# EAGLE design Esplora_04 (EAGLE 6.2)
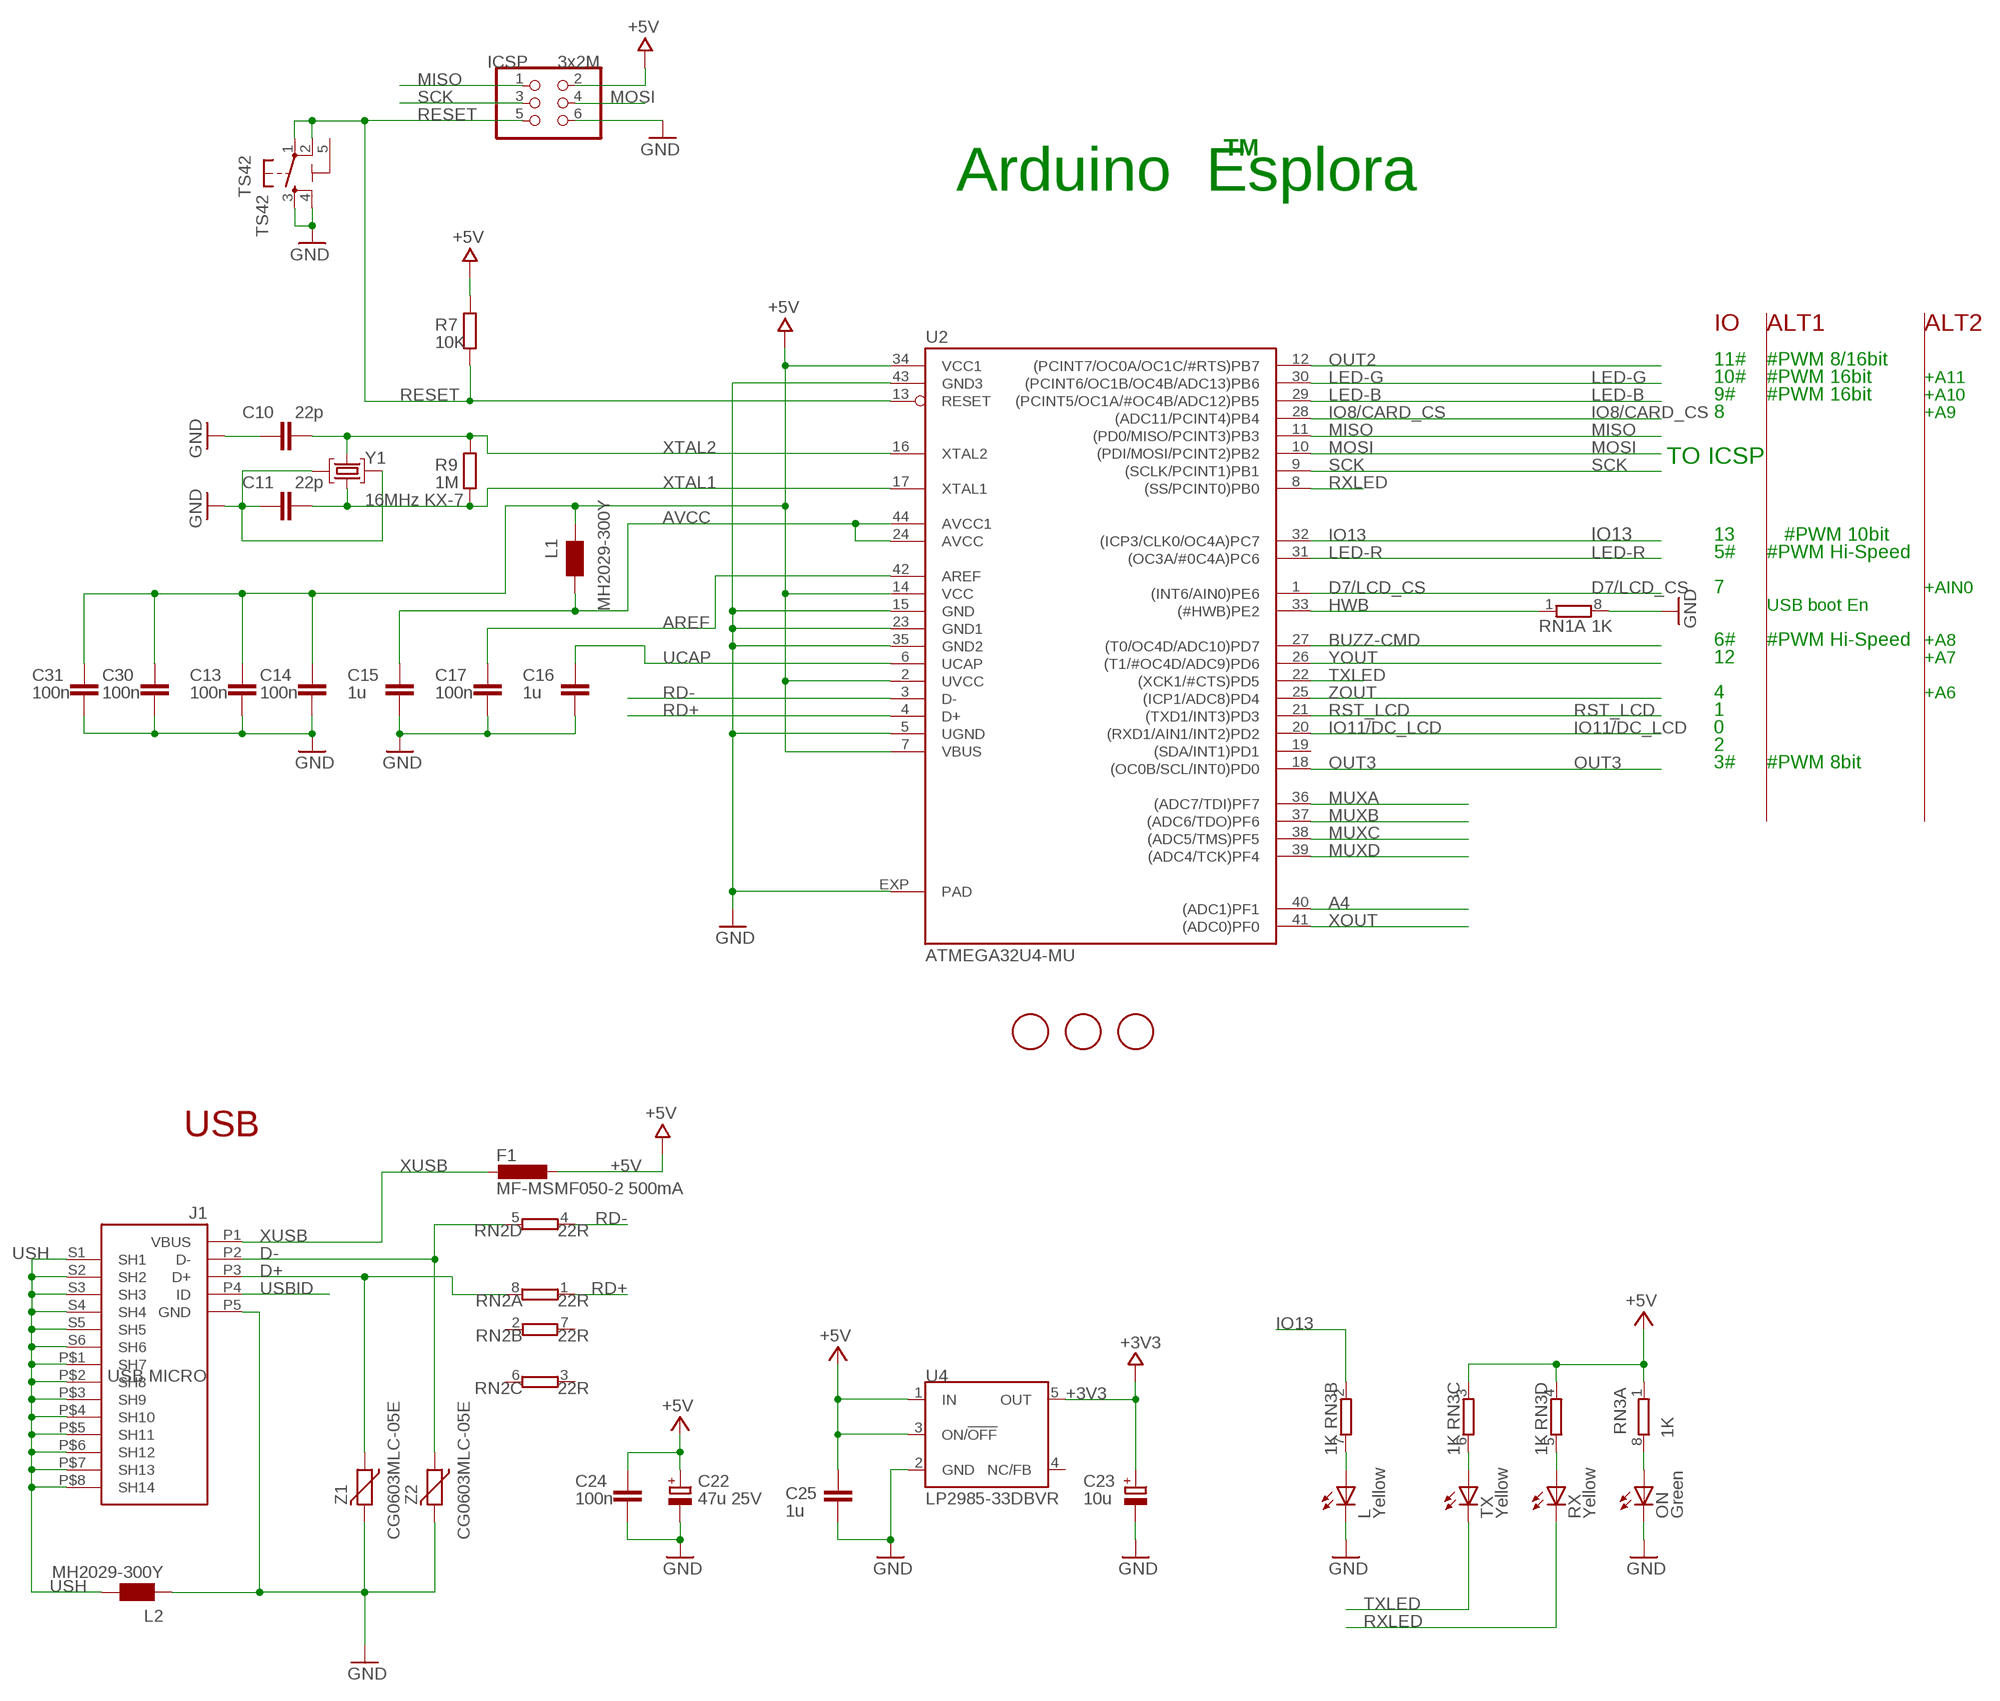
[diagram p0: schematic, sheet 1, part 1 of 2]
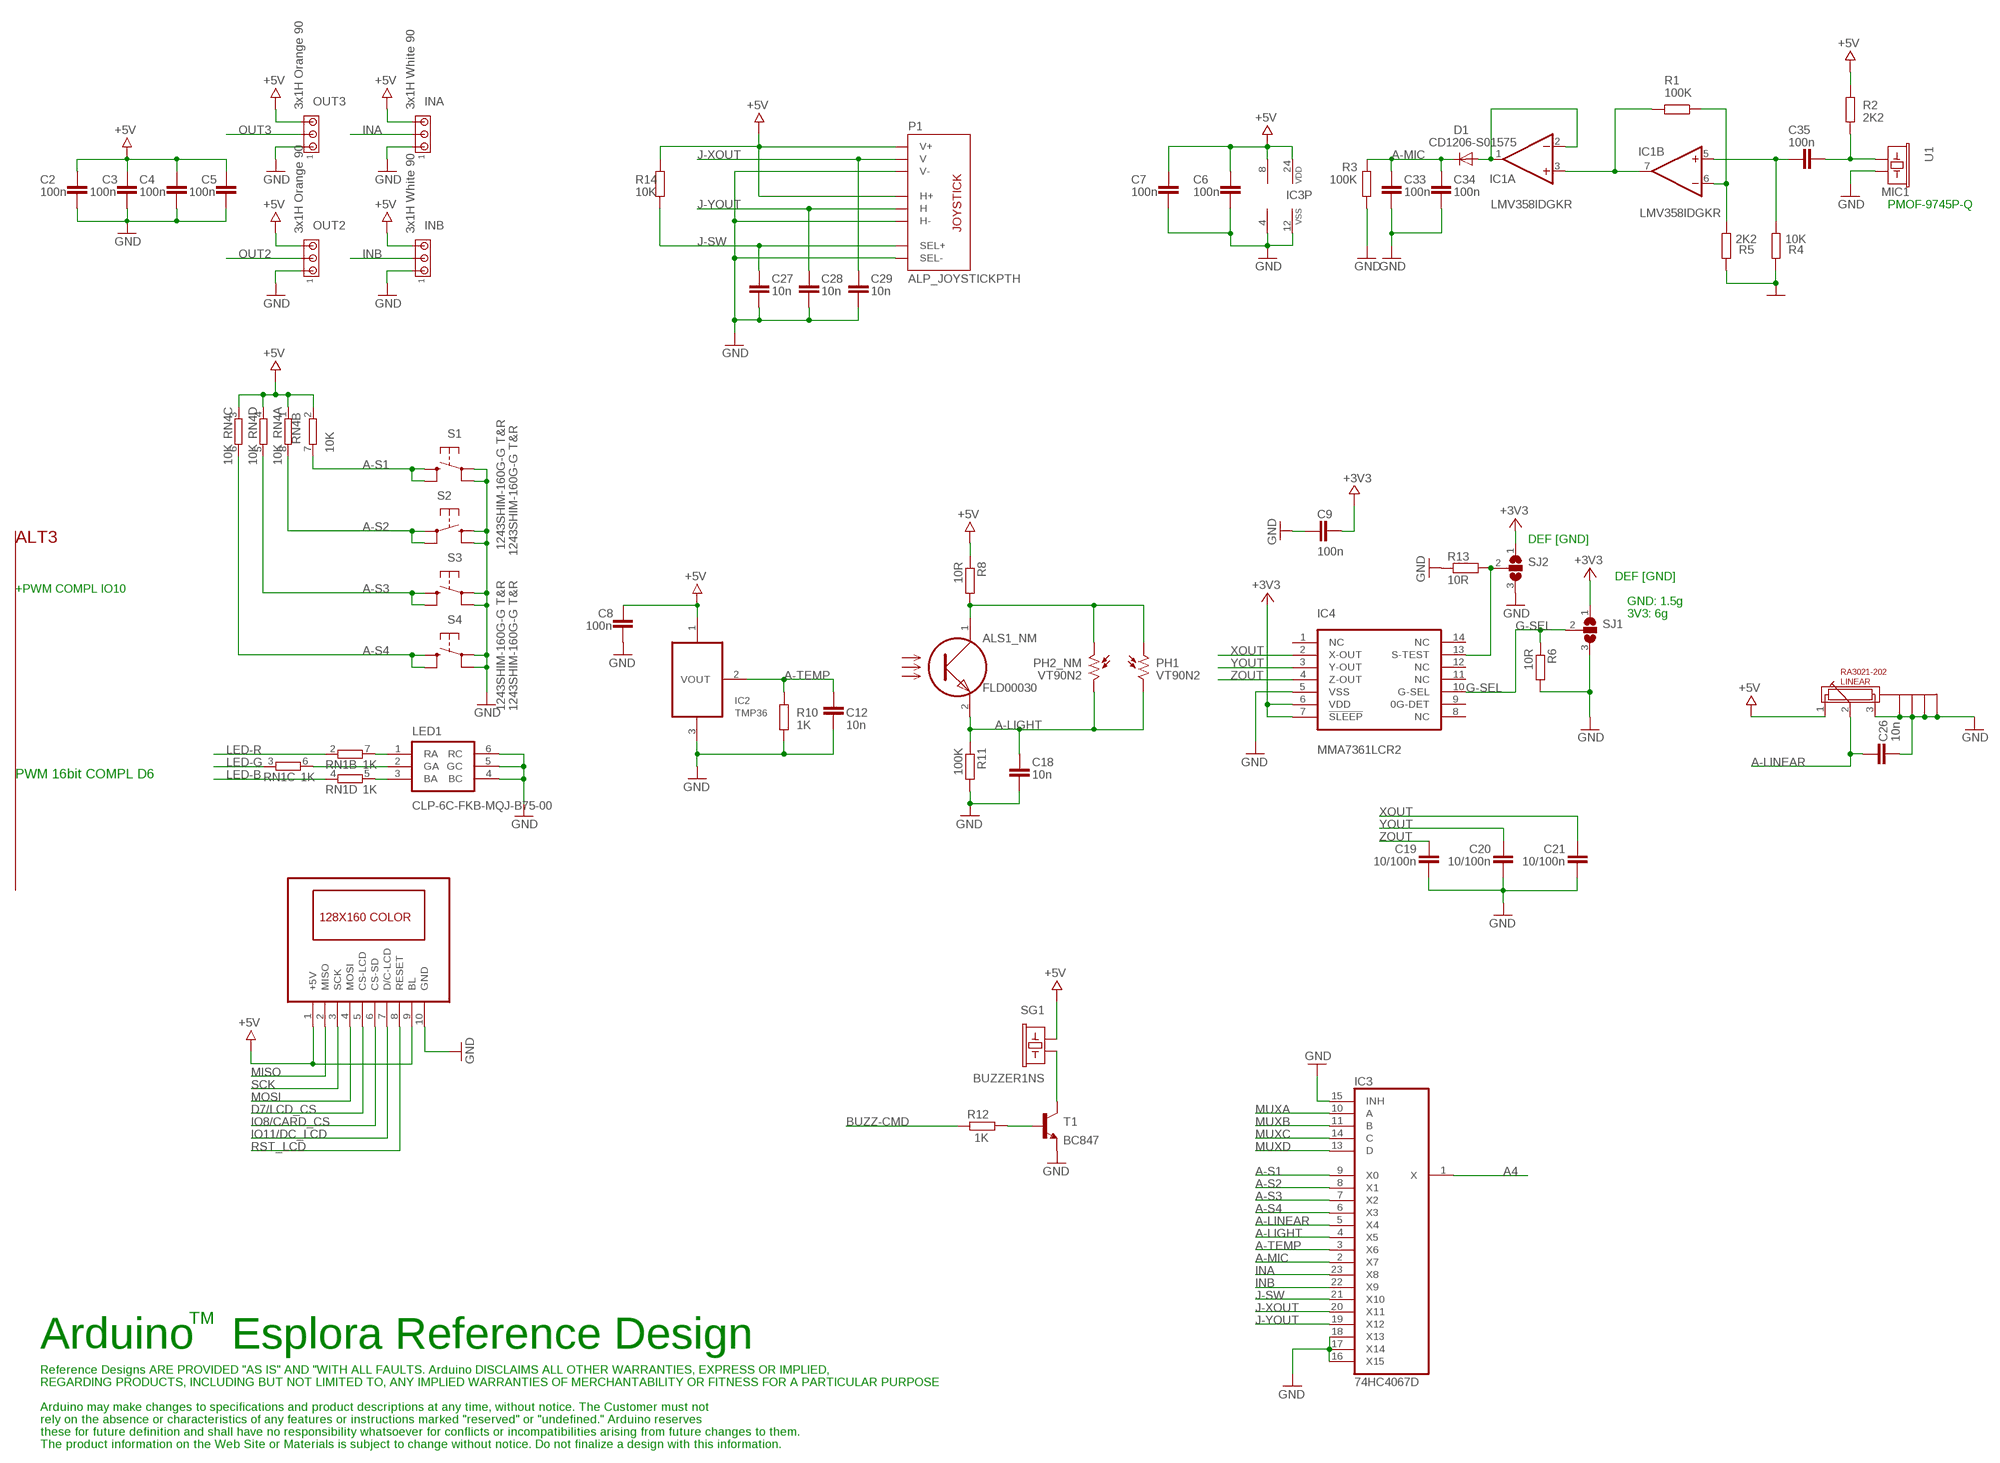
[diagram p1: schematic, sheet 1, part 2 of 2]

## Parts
ALS1_NM  FLD00030  [FLD00030]
C2  100n  C-EUC0603  [C0603-ROUND]
C3  100n  C-EUC0603  [C0603-ROUND]
C4  100n  C-EUC0603  [C0603-ROUND]
C5  100n  C-EUC0603  [C0603-ROUND]
C6  100n  C-EUC0603  [C0603-ROUND]
C7  100n  C-EUC0603  [C0603-ROUND]
C8  100n  C-EUC0603  [C0603-ROUND]
C9  100n  C-EUC0603  [C0603-ROUND]
C10  22p  C-EUC0603  [C0603-ROUND]
C11  22p  C-EUC0603  [C0603-ROUND]
C12  10n  C-EUC0603  [C0603-ROUND]
C13  100n  C-EUC0603  [C0603-ROUND]
C14  100n  C-EUC0603  [C0603-ROUND]
C15  1u  C-EUC0603  [C0603-ROUND]
C16  1u  C-EUC0603  [C0603-ROUND]
C17  100n  C-EUC0603  [C0603-ROUND]
C18  10n  C-EUC0603  [C0603-ROUND]
C19  10/100n  C-EUC0603  [C0603-ROUND]
C20  10/100n  C-EUC0603  [C0603-ROUND]
C21  10/100n  C-EUC0603  [C0603-ROUND]
C22  47u 25V  CPOL-EUD  [PANASONIC_D]
C23  10u  CPOL-EUSMCB  [SMC_B]
C24  100n  C-EUC0603  [C0603-ROUND]
C25  1u  C-EUC0603  [C0603-ROUND]
C26  10n  C-EUC0603  [C0603-ROUND]
C27  10n  C-EUC0603  [C0603-ROUND]
C28  10n  C-EUC0603  [C0603-ROUND]
C29  10n  C-EUC0603  [C0603-ROUND]
C30  100n  C-EUC0603  [C0603-ROUND]
C31  100n  C-EUC0603  [C0603-ROUND]
C33  100n  C-EUC0603  [C0603-ROUND]
C34  100n  C-EUC0603  [C0603-ROUND]
C35  100n  C-EUC0603  [C0603-ROUND]
D1  CD1206-S01575  DIODE-MINIMELF  [MINIMELF]
F1  MF-MSMF050-2 500mA  L-EUL1812  [L1812]
FID1  FIDUCIALMOUNT  [FIDUCIA-MOUNT]
FID2  FIDUCIALMOUNT  [FIDUCIA-MOUNT]
FID3  FIDUCIALMOUNT  [FIDUCIA-MOUNT]
IC1  LMV358IDGKR  LMV358MMX  [MSOP08]
IC2  TMP36  LM35TO-92  [TO92]
IC3  74HC4067D  4067D  [SO24W]
IC4  MMA7361LCR2  MMA7361LC  [LGA-14_3X5/0.8]
ICSP  3x2M  PINHD-2X3  [2X03]
INA  3x1H White 90  MTA03-100  [10X03MTA]
INB  3x1H White 90  MTA03-100  [10X03MTA]
J1  USB MICRO  MYCON2_USB-MINI-B  [CON2_USB_MICRO_B_AT]
L  Yellow  LEDCHIPLED_0805  [CHIPLED_0805]
L1  MH2029-300Y  WE-CBF_0805  [0805]
L2  MH2029-300Y  WE-CBF_0805  [0805]
LCD1  LCD1  1.8'_LCD-TFT(128X160)+SD-CARD  [1.8'_LCD-LCD-TFT(128X160)]
LED1  CLP-6C-FKB-MQJ-B75-00  RGB-LED  [RGB-LED]
LINEAR  RA3021-202  [RA3021-202]
ON  Green  LEDCHIPLED_0805  [CHIPLED_0805]
OUT2  3x1H Orange 90  MTA03-100  [10X03MTA]
OUT3  3x1H Orange 90  MTA03-100  [10X03MTA]
P1  ALP_JOYSTICKPTH  [ALP_JOYSTICK]
PH1  VT90N2  A1050_09  [T0-46-A10XX]
PH2_NM  VT90N2  B1060_23  [TO-8_B10]
R1  100K  R-EU_R0603  [R0603-ROUND]
R2  2K2  R-EU_R0603  [R0603-ROUND]
R3  100K  R-EU_R0603  [R0603-ROUND]
R4  10K  R-EU_R0603  [R0603-ROUND]
R5  2K2  R-EU_R0603  [R0603-ROUND]
R6  10R  R-EU_R0603  [R0603-ROUND]
R7  10K  R-EU_R0603  [R0603-ROUND]
R8  10R  R-EU_R0603  [R0603-ROUND]
R9  1M  R-EU_R0603  [R0603-ROUND]
R10  1K  R-EU_R0603  [R0603-ROUND]
R11  100K  R-EU_R0603  [R0603-ROUND]
R12  1K  R-EU_R0603  [R0603-ROUND]
R13  10R  R-EU_R0603  [R0603-ROUND]
R14  10K  R-EU_R1206  [R1206]
RN1  1K  4R-NCAY16  [CAY16]
RN2  22R  4R-NCAY16  [CAY16]
RN3  1K  4R-NCAY16  [CAY16]
RN4  10K  4R-NCAY16  [CAY16]
RX  Yellow  LEDCHIPLED_0805  [CHIPLED_0805]
S1  1243SHIM-160G-G T&R  TACTILE_SWITCHTACTILE_SWITCH_SMD-12MM  [TACTILE-SMD-12MM]
S2  1243SHIM-160G-G T&R  TACTILE_SWITCHTACTILE_SWITCH_SMD-12MM  [TACTILE-SMD-12MM]
S3  1243SHIM-160G-G T&R  TACTILE_SWITCHTACTILE_SWITCH_SMD-12MM  [TACTILE-SMD-12MM]
S4  1243SHIM-160G-G T&R  TACTILE_SWITCHTACTILE_SWITCH_SMD-12MM  [TACTILE-SMD-12MM]
SG1  BUZZER1NS  [BUZZER-12MM-NS]
SJ1  SJ2W  [SJ_2]
SJ2  SJ2W  [SJ_2]
T1  BC847  [SOT23]
TS42  TS42  [TS42]
TX  Yellow  LEDCHIPLED_0805  [CHIPLED_0805]
U1  MIC1  MIC9.7MM  [MIC-9.7MM]
U2  ATMEGA32U4-MU  [QFN44ML7X7]
U4  LP2985-33DBVR  LP2985-XXDBVR33  [SOT23-DBV]
Y1  16MHz KX-7  CRYSTAL-3.2-2.5  [CRYSTAL-3.2-2.5]
Z1  CG0603MLC-05E  VARISTORCN0603  [CT/CN0603]
Z2  CG0603MLC-05E  VARISTORCN0603  [CT/CN0603]

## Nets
+3V3 [power]: C9.2 C23.+ IC4.6(VDD) IC4.7(!SLEEP) SJ1.1 SJ2.1 U4.5(OUT)
+5V [power]: C2.2 C3.2 C4.2 C5.2 C6.2 C7.2 C8.2 C13.1 C14.1 C22.+ C24.2 C25.2 C30.1 C31.1 F1.1 IC1.8(P:V+) IC2.1(+VS) IC3.24(VDD) ICSP.2 INA.3 INB.3 L1.1 LCD1.1(+5V) LCD1.9(BL) LINEAR.1 OUT2.3 OUT3.3 P1.H1(H+) P1.V1(V+) R2.1 R7.1 R8.1 R14.1 RN3.1 RN3.3 RN3.4 RN4.1 RN4.2 RN4.3 RN4.4 SG1.+ U2.2(UVCC) U2.7(VBUS) U2.14(VCC) U2.34(VCC1) U4.1(IN) U4.3(ON/!OFF)
A4: IC3.1(X) U2.40((ADC1)PF1)
A-LIGHT: ALS1_NM.2 C18.2 IC3.4(X5) PH1.2 PH2_NM.2 R11.1
A-LINEAR: C26.2 IC3.5(X4) LINEAR.2
A-MIC: C33.2 C34.2 D1.C IC3.2(X7) R3.1
A-S1: IC3.9(X0) RN4.7 S1.P$3 S1.P$4
A-S2: IC3.8(X1) RN4.8 S2.P$1 S2.P$2
A-S3: IC3.7(X2) RN4.5 S3.P$3 S3.P$4
A-S4: IC3.6(X3) RN4.6 S4.P$3 S4.P$4
A-TEMP: C12.2 IC2.2(VOUT) IC3.3(X6) R10.1
AREF [aref]: C17.2 U2.42(AREF)
AVCC: C15.1 L1.2 U2.24(AVCC) U2.44(AVCC1)
BUZZ-CMD: R12.2 U2.27((T0/OC4D/ADC10)PD7)
D7/LCD_CS: LCD1.5(CS-LCD) U2.1((INT6/AIN0)PE6)
D+: J1.P3(D+) RN2.8 Z1.1
D-: J1.P2(D-) RN2.5 Z2.1
G-SEL: IC4.10(G-SEL) R6.1 SJ1.2
GND [gnd]: C2.1 C3.1 C4.1 C5.1 C6.1 C7.1 C8.1 C9.1 C10.1 C11.2 C12.1 C13.2 C14.2 C15.2 C16.2 C17.1 C18.1 C19.1 C20.1 C21.1 C22.- C23.- C24.1 C25.1 C26.1 C27.1 C28.1 C29.1 C30.2 C31.2 C33.1 C34.1 IC1.4(P:V-) IC2.3(GND) IC3.12(VSS) IC3.15(INH) IC3.16(X15) IC3.17(X14) IC3.18(X13) IC4.5(VSS) ICSP.6 INA.1 INB.1 J1.P5(GND) L2.1 L.C LCD1.10(GND) LED1.4(BC) LED1.5(GC) LED1.6(RC) LINEAR.3 LINEAR.CHASSIS1(CHASSIS-GND-1) LINEAR.CHASSIS2(CHASSIS-GND-2) LINEAR.CHASSIS3(CHASSIS-GND-3) LINEAR.CHASSIS4(CHASSIS-GND-4) ON.C OUT2.1 OUT3.1 P1.B2A(SEL-) P1.H3(H-) P1.V3(V-) R3.2 R4.2 R5.2 R6.2 R10.2 R11.2 R13.1 RN1.8 S1.P$1 S1.P$2 S2.P$3 S2.P$4 S3.P$1 S3.P$2 S4.P$1 S4.P$2 SJ1.3 SJ2.3 T1.2(E) TS42.3 TS42.4 U1.2 U2.5(UGND) U2.15(GND) U2.23(GND1) U2.35(GND2) U2.43(GND3) U2.EXP(PAD) U4.2(GND) Y1.2(GND) Y1.4(GND) Z1.2 Z2.2
HWB: RN1.1 U2.33((#HWB)PE2)
INA: IC3.23(X8) INA.2
INB: IC3.22(X9) INB.2
IO8/CARD_CS: LCD1.6(CS-SD) U2.28((ADC11/PCINT4)PB4)
IO11/DC_LCD: LCD1.7(D/C-LCD) U2.20((RXD1/AIN1/INT2)PD2)
IO13: RN3.2 U2.32((ICP3/CLK0/OC4A)PC7)
J-SW: C27.2 IC3.21(X10) P1.B1A(SEL+) R14.2
J-XOUT: C29.2 IC3.20(X11) P1.V2(V)
J-YOUT: C28.2 IC3.19(X12) P1.H2(H)
LED-B: RN1.4 U2.29((PCINT5/OC1A/#OC4B/ADC12)PB5)
LED-G: RN1.3 U2.30((PCINT6/OC1B/OC4B/ADC13)PB6)
LED-R: RN1.2 U2.31((OC3A/#0C4A)PC6)
MISO: ICSP.1 LCD1.2(MISO) U2.11((PD0/MISO/PCINT3)PB3)
MOSI: ICSP.4 LCD1.4(MOSI) U2.10((PDI/MOSI/PCINT2)PB2)
MUXA: IC3.10(A) U2.36((ADC7/TDI)PF7)
MUXB: IC3.11(B) U2.37((ADC6/TDO)PF6)
MUXC: IC3.14(C) U2.38((ADC5/TMS)PF5)
MUXD: IC3.13(D) U2.39((ADC4/TCK)PF4)
N$1: D1.A IC1.1(A:OUT) IC1.2(A:-IN)
N$2: L.A RN3.7
N$3: ON.A RN3.8
N$4: IC4.13(S-TEST) R13.2 SJ2.2
N$6: RN3.6 TX.A
N$8: RN3.5 RX.A
N$11: LED1.1(RA) RN1.7
N$12: LED1.2(GA) RN1.6
N$13: LED1.3(BA) RN1.5
N$17: SG1.- T1.3(C)
N$19: C35.1 R2.2 U1.1
N$20: C35.2 IC1.5(B:+IN) R4.1
N$21: IC1.6(B:-IN) R1.1 R5.1
N$23: IC1.3(A:+IN) IC1.7(B:OUT) R1.2
N$27: ALS1_NM.1 PH1.1 PH2_NM.1 R8.2
N$31: R12.1 T1.1(B)
OUT2: OUT2.2 U2.12((PCINT7/OC0A/OC1C/#RTS)PB7)
OUT3: OUT3.2 U2.18((OC0B/SCL/INT0)PD0)
RD+: RN2.1 U2.4(D+)
RD-: RN2.4 U2.3(D-)
RESET: ICSP.5 R7.2 TS42.1 TS42.2 U2.13(RESET)
RST_LCD: LCD1.8(RESET) U2.21((TXD1/INT3)PD3)
RXLED: RX.C U2.8((SS/PCINT0)PB0)
SCK: ICSP.3 LCD1.3(SCK) U2.9((SCLK/PCINT1)PB1)
TXLED: TX.C U2.22((XCK1/#CTS)PD5)
UCAP: C16.1 U2.6(UCAP)
USBID: J1.P4(ID)
USH [gnd]: J1.P$1(SH7) J1.P$2(SH8) J1.P$3(SH9) J1.P$4(SH10) J1.P$5(SH11) J1.P$6(SH12) J1.P$7(SH13) J1.P$8(SH14) J1.S1(SH1) J1.S2(SH2) J1.S3(SH3) J1.S4(SH4) J1.S5(SH5) J1.S6(SH6) L2.2
XOUT: C21.2 IC4.2(X-OUT) U2.41((ADC0)PF0)
XTAL1: C11.1 R9.1 U2.17(XTAL1) Y1.1(C1)
XTAL2: C10.2 R9.2 U2.16(XTAL2) Y1.3(C2)
XUSB [usbvcc]: F1.2 J1.P1(VBUS)
YOUT: C20.2 IC4.3(Y-OUT) U2.26((T1/#OC4D/ADC9)PD6)
ZOUT: C19.2 IC4.4(Z-OUT) U2.25((ICP1/ADC8)PD4)
Unconnected: IC4.1(NC) IC4.8(NC) IC4.9(0G-DET) IC4.11(NC) IC4.12(NC) IC4.14(NC) RN2.2 RN2.3 RN2.6 RN2.7 U2.19((SDA/INT1)PD1) U4.4(NC/FB)

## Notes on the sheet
- PMOF-9745P-Q
- TM
- Arduino  Esplora
- IO | ALT1 | ALT2 | ALT3 | DEF [GND]
- 11# | #PWM 8/16bit
- 10# | #PWM 16bit | +A11 | DEF [GND]
- 9# | #PWM 16bit | +A10 | +PWM COMPL IO10
- 8 | +A9 | GND: 1.5g
- 3V3: 6g
- TO ICSP
- 13 | #PWM 10bit
- 5# | #PWM Hi-Speed
- 7 | +AIN0
- USB boot En
- 6# | #PWM Hi-Speed | +A8
- 12 | +A7 | PWM 16bit COMPL D6
- 4 | +A6
- 1
- 0
- 2
- 3# | #PWM 8bit
- USB
- TM
- Arduino   Esplora Reference Design
- Reference Designs ARE PROVIDED "AS IS" AND "WITH ALL FAULTS. Arduino DISCLAIMS ALL OTHER WARRANTIES, EXPRESS OR IMPLIED,
- REGARDING PRODUCTS, INCLUDING BUT NOT LIMITED TO, ANY IMPLIED WARRANTIES OF MERCHANTABILITY OR FITNESS FOR A PARTICULAR PURPOSE
- Arduino may make changes to specifications and product descriptions at any time, without notice. The Customer must not
- rely on the absence or characteristics of any features or instructions marked "reserved" or "undefined." Arduino reserves
- these for future definition and shall have no responsibility whatsoever for conflicts or incompatibilities arising from future changes to them.
- The product information on the Web Site or Materials is subject to change without notice. Do not finalize a design with this information.

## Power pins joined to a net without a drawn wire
5-GND: TS42.5(5-GND)

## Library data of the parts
ALS1_NM = SmartPrj:FLD00030: FLD00030 Analog Ambient Light Sensor FAIRCHILD Semiconductor
C2-C21 C24-C31 C33-C35 = SmartPrj:C-EU: CAPACITOR, European symbol
C22 C23 = rcl:CPOL-EU: POLARIZED CAPACITOR, European symbol
D1 = diode:DIODE-: DIODE
F1 = rcl:L-EU: INDUCTOR, European symbol
FID1-FID3 = SmartPrj:FIDUCIALMOUNT
IC1 = linear:LMV358?*: Dual General Purpose, Low Voltage, Rail-to-Rail Output Operational Amplifiers Source: http://www.national.com/mpf/LM/LMV321.html http://www.national.com/dt/lmv_qual.pdf
IC2 = SmartPrj:LM35: LM35 Precision Centigrade Temperature Sensors
IC3 = 40xx:4067: 16-channel ANALOG MULTIPLEXER
IC4 = SmartPrj:MMA7361LC: MMA7361LC Three Axis Accelerometer Freescale Semiconductor
ICSP = SmartPrj:PINHD-2X3: PIN HEADER
INA INB OUT2 OUT3 = con-amp:MTA03-100: AMP connector
J1 = SmartPrj:MYCON2_USB-MINI-B
L ON RX TX = led:LED: LED
L1 L2 = wuerth-elektronik:WE-CBF: SMD EMI Suppression Ferrite Beads
LCD1 = SmartPrj:1.8'_LCD-TFT(128X160)+SD-CARD: 1.8Inch LCD Display + SD Card SmartProjects.it
LED1 = SmartPrj:RGB-LED: CREE RGB-LED/PLCC6-SMD
LINEAR = st-mod v1.1:RA3021-202: RA3021-202 Linear Potentiometer P.C.B. single unit case-earthing mounting type Travel: 30mm
P1 = tinker_it:ALP_JOYSTICK: Thumb Joystick Joystick commonly found in PS2 controllers. Two pots and a select switch. Footprint proven. Spark Fun Electronics SKU : COM-09032
PH1 = photo-elements:A10: Sensor Robust Light Sensing Applications
PH2_NM = photo-elements:?1060*: Sensor Street Light control
R1-R14 = SmartPrj:R-EU_: RESISTOR, European symbol
RN1-RN4 = resistor-dil:4R-N: Array Chip Resistor Source: RS Component / Phycomp; OC_FARNELL: unknown; OC_NEWARK: unknown
S1-S4 = SmartPrj:TACTILE_SWITCH: Momentary Switch Button commonly used for reset or general input.
SG1 = SmartPrj:BUZZER1: Buzzer 12-22mm
SJ1 SJ2 = jumper:SJ2W: SMD solder JUMPER
T1 = transistor:BC847: NPN TRANSISTOR
TS42 = SmartPrj:TS42: TS42 Dongnan Electronics Tact switch VDC 12V - 50mA
U1 = SparkFun:MIC: Microphone
U2 = SmartPrj:ATMEGA32U4-
U4 = SmartPrj:LP2985-XXDBVR: ULTRALOW-POWER 50-mA LOW-DROPOUT LINEAR REGULATORS 50-mA Low-Dropout Regulator Source: http://focus.ti.com/lit/ds/symlink/tps77001.pdf
Y1 = SmartPrj:CRYSTAL-3.2-2.5
Z1 Z2 = varistor:VARISTOR: VARISTOR

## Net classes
0 default: width 0.254 mm, drill 0.61 mm, clearance 0.254 mm
1 power: width 0.254 mm, drill 0.61 mm, clearance 0.254 mm
2 gnd: width 0.254 mm, drill 0.61 mm, clearance 0.254 mm
3 usbvcc: width 0.254 mm, drill 0.61 mm, clearance 0.254 mm
4 aref: width 0.254 mm, drill 0.61 mm, clearance 0.254 mm

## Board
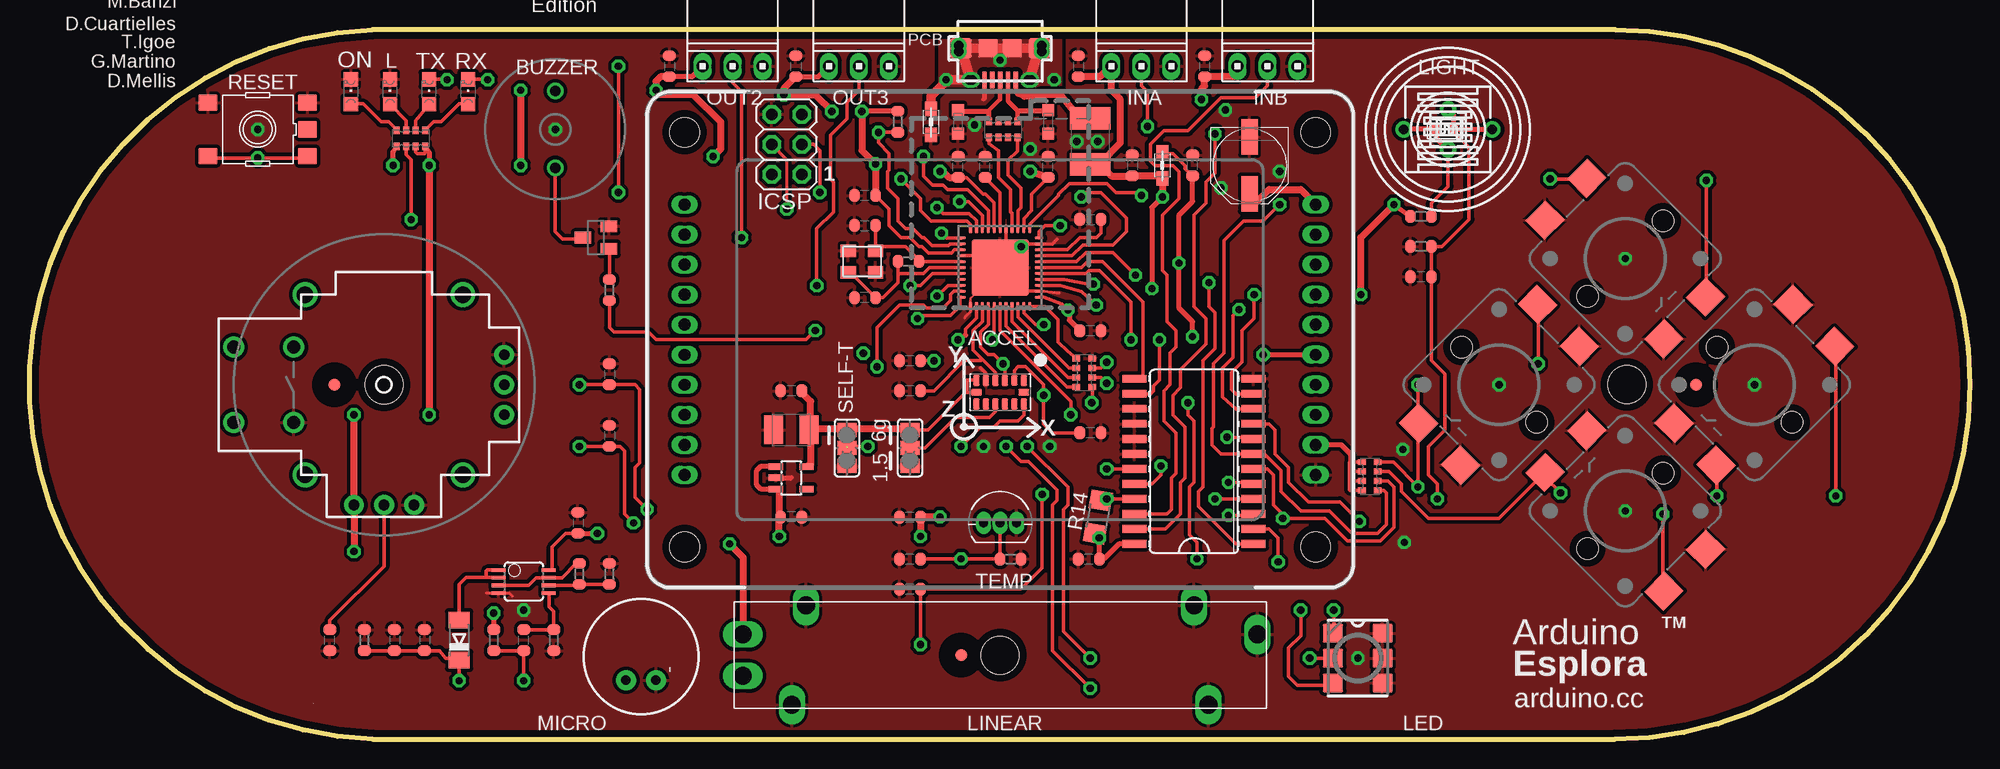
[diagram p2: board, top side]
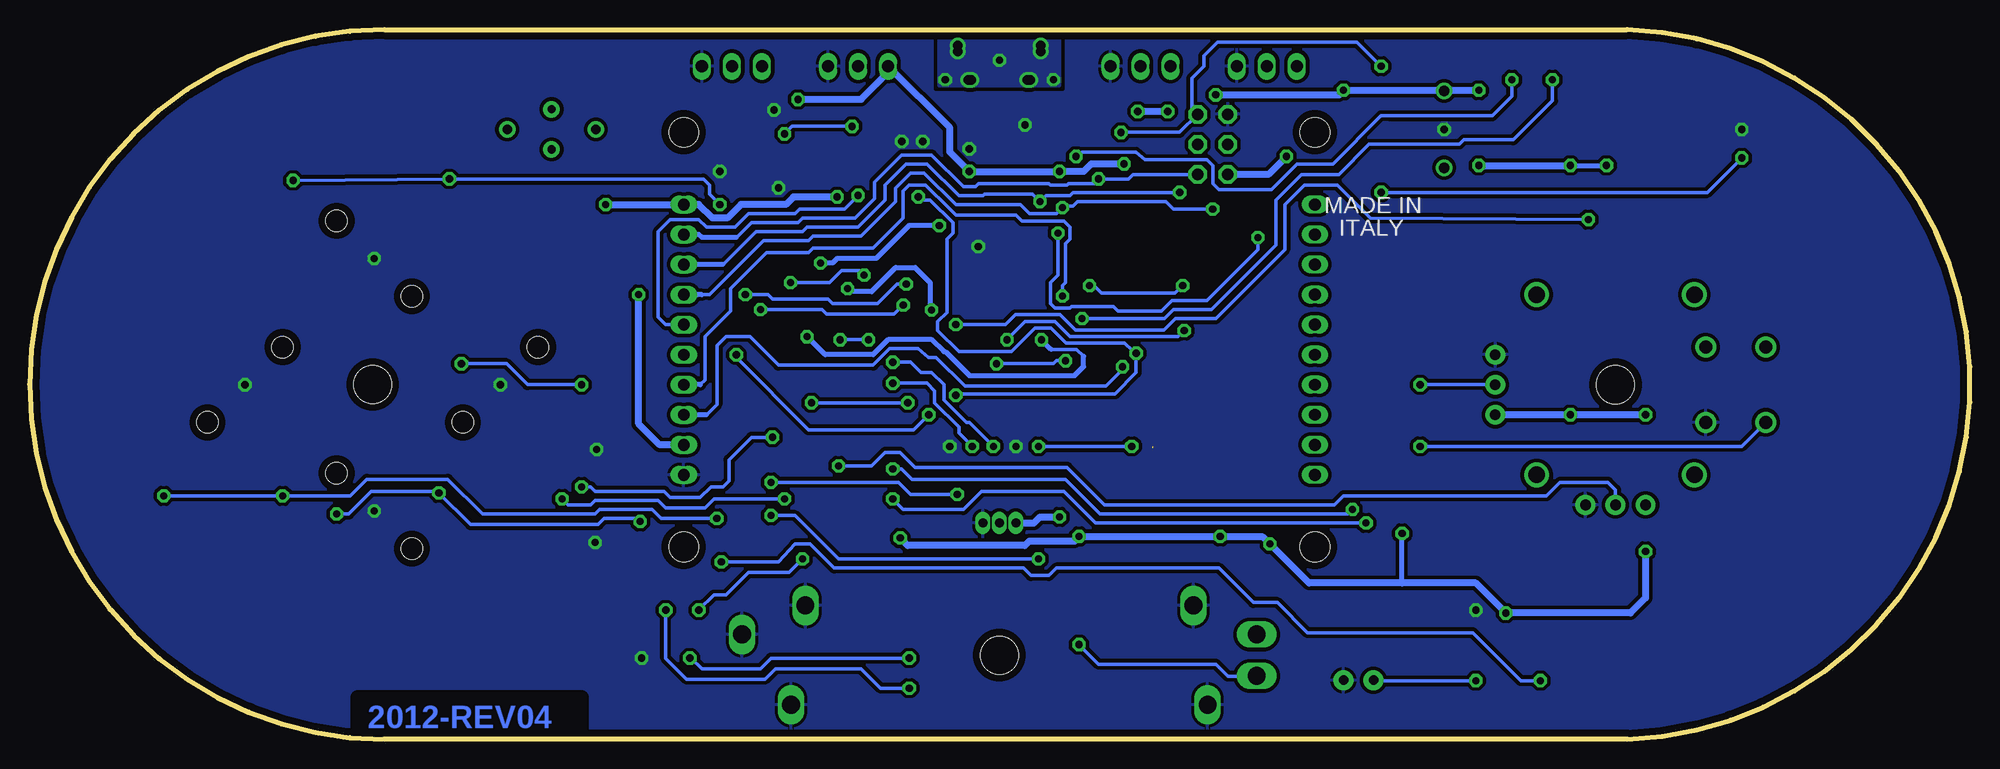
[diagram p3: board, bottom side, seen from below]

Size 163.98 x 60 mm. Coordinates in mm from the lower left corner, seen from the top.
Outline: 28.98,0 133.98,0 arc180 133.98,60 28.98,60 arc176 28.98,0
Copper layers (1*16): Top 0.035mm / dielectric 1.5mm / Bottom 0.035mm
Design rules: minimum track width 10mil, minimum drill 22mil, track to track 10mil, track to pad 10mil, pad to pad 8mil, via to via 12mil, smd to smd 8mil, copper to edge 24mil, drill to drill 12mil, minimum pad ring 10mil, minimum via ring 10mil, stop-mask expansion 2mil, vias tented up to drill 30mil, thermal gap 10mil
Holes 3.2 mm at 82.02,7.11 29.95,29.97 134.98,30
bRestrict: 3 lines
vRestrict: area 47.9,10.3 to 48.5,10.8; area 50.4,10.2 to 50.9,11

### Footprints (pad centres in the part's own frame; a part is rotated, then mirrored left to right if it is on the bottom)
FLD00030 = smd 0.8 x 0.9: 1 -0.75,0; 2 0.75,0
C0603-ROUND = smd 0.898 x 1.1: 1 -0.889,0; 2 0.889,0
PANASONIC_D = smd 3 x 1.4: + 2.4,0; - -2.4,0
SMC_B = smd 1.6 x 2.4: + -1.5,0; - 1.5,0
MINIMELF = smd 1.4 x 1.8: A 1.7,0; C -1.7,0
L1812 = smd 1.9 x 3.4: 1 -1.95,0; 2 1.95,0
FIDUCIA-MOUNT = smd 1.016 x 1.016: P$1 0,0
MSOP08 = smd 0.3 x 1.2: 1 -0.976,-2.113; 2 -0.326,-2.113; 3 0.324,-2.113; 4 0.974,-2.113; 5 0.974,2.112; 6 0.324,2.112; 7 -0.326,2.112; 8 -0.976,2.112
TO92 = drill 0.75 pad 1.092 long: 1 -1.397,0; 2 0,0; 3 1.397,0
SO24W = smd 0.66 x 2.032: 1 -6.985,-5.029; 2 -5.715,-5.029; 3 -4.445,-5.029; 4 -3.175,-5.029; 5 -1.905,-5.029; 6 -0.635,-5.029; 7 0.635,-5.029; 8 1.905,-5.029; 9 3.175,-5.029; 10 4.445,-5.029; 11 5.715,-5.029; 12 6.985,-5.029; 13 6.985,5.029; 14 5.715,5.029; 15 4.445,5.029; 16 3.175,5.029; 17 1.905,5.029; 18 0.635,5.029; 19 -0.635,5.029; 20 -1.905,5.029; 21 -3.175,5.029; 22 -4.445,5.029; 23 -5.715,5.029; 24 -6.985,5.029
LGA-14_3X5/0.8 = smd 0.55 x 0.9: 1 -2,-1; 3 -0.4,-1; 4 0.4,-1; 5 1.2,-1; 6 2,-1; 8 2,1; 9 1.2,1; 10 0.4,1; 11 -0.4,1; 12 -1.2,1; 13 -2,1 | smd 0.55 x 0.85: 2 -1.2,-1 | smd 0.9 x 0.55: 7 2,0; 14 -2,0
2X03 = drill 0.95 pad 1.55 octagon: 1 -2.54,-1.27; 2 -2.54,1.27; 3 0,-1.27; 4 0,1.27; 5 2.54,-1.27; 6 2.54,1.27
10X03MTA = drill 1.016 long: 1 2.54,0; 2 0,0; 3 -2.54,0
CON2_USB_MICRO_B_AT = smd 0.406 x 1.346: P1 -1.321,2.692; P2 -0.66,2.692; P3 0,2.692; P4 0.66,2.692; P5 1.321,2.692 | drill 0.8 pad 1.27: P$1 -2.616,2.692 | drill 0.8 pad 1.245: P$2 -2.362,2.692; P$7 2.362,2.692; P$8 2.616,2.692 | drill 0.8 pad 1.143: P$3 -3.505,-0.254; P$4 -3.505,0.254; P$5 3.505,0.254; P$6 3.505,-0.254 | smd 1.778 x 1.651: S1 -3.302,0; S2 3.302,0 | smd 1.524 x 1.27: S3 -2.489,2.692; S4 2.489,2.692 | smd 1.626 x 1.524: S5 -1.016,0; S6 1.016,0
CHIPLED_0805 = smd 1.2 x 1.2: A 0,-1.05; C 0,1.05
0805 = smd 1.2 x 1: 1 -1.1,0; 2 1.1,0
1.8'_LCD-LCD-TFT(128X160) = drill 1 long: 1 11.43,-26.67; 2 8.89,-26.67; 3 6.35,-26.67; 4 3.81,-26.67; 5 1.27,-26.67; 6 -1.27,-26.67; 7 -3.81,-26.67; 8 -6.35,-26.67; 9 -8.89,-26.67; 10 -11.43,-26.67; 11 11.43,26.67; 12 8.89,26.67; 13 6.35,26.67; 14 3.81,26.67; 15 1.27,26.67; 16 -1.27,26.67; 17 -3.81,26.67; 18 -6.35,26.67; 19 -8.89,26.67; 20 -11.43,26.67 | hole 2.5: -17.526,-26.67; 17.526,-26.67; 17.526,26.67; -17.526,26.67
RGB-LED = smd 1.7 x 1.55: 1 -2.1,2.1; 2 -2.1,0; 3 -2.1,-2.1; 4 2.1,-2.1; 5 2.1,0; 6 2.1,2.1
RA3021-202 = drill 1.5 long: 1 -21.75,1.75; 2 -21.75,-1.75; 3 21.75,1.75; CHASSIS1 -16.4,4.2; CHASSIS2 16.4,4.2; CHASSIS3 -17.6,-4.2; CHASSIS4 17.6,-4.2
ALP_JOYSTICK = drill 1.1 pad 1.778: B1A -3.175,12.7; B1B 3.175,12.7; B2A -3.175,7.62; B2B 3.175,7.62 | drill 0.889 pad 1.676: H1 -2.54,-10.16; H2 0,-10.16; H3 2.54,-10.16; V1 -10.16,2.54; V2 -10.16,0; V3 -10.16,-2.54 | drill 1.397: MOUNT1 -7.62,6.668; MOUNT2 -7.62,-6.668; MOUNT3 7.62,-6.668; MOUNT4 7.62,6.668
T0-46-A10XX = drill 0.7 pad 1.4: 1 -1.7,0; 2 1.7,0
TO-8_B10 = drill 0.8 pad 1.4: 1 -3.75,0; 2 3.75,0
R0603-ROUND = smd 0.898 x 1.1: 1 -0.889,0; 2 0.889,0
R1206 = smd 1.6 x 1.803: 1 -1.422,0; 2 1.422,0
CAY16 = smd 0.5 x 0.65: 1 -1.2,-0.675; 2 -0.4,-0.675; 3 0.4,-0.675; 4 1.2,-0.675; 5 1.2,0.675; 6 0.4,0.675; 7 -0.4,0.675; 8 -1.2,0.675
TACTILE-SMD-12MM = smd 2.3 x 2.4: P$1 7.1,-2.5; P$2 -7.1,-2.5; P$3 7.1,2.5; P$4 -7.1,2.5 | hole 1.8: 0,4.5; 0,-4.5
BUZZER-12MM-NS = drill 0.9: + 3.25,0; - -3.25,0
SJ_2 = smd 1.168 x 1.6: 1 -1.524,0; 2 0,0; 3 1.524,0
SOT23 = smd 1 x 1.4: 1 -0.95,-1.1; 2 0.95,-1.1; 3 0,1.1
TS42 = smd 1.6 x 1.4: 1 -4.2,2.25; 2 4.2,2.25; 3 -4.2,-2.25; 4 4.2,-2.25; 5 -4.2,0
MIC-9.7MM = drill 0.8 pad 1.676: 1 -2,1.27; 2 -2,-1.27
QFN44ML7X7 = smd 0.75 x 0.275: 1 -3.275,2.5; 2 -3.275,2; 3 -3.275,1.5; 4 -3.275,1; 5 -3.275,0.5; 6 -3.275,0; 7 -3.275,-0.5; 8 -3.275,-1; 9 -3.275,-1.5; 10 -3.275,-2; 11 -3.275,-2.5; 23 3.275,-2.5; 24 3.275,-2; 25 3.275,-1.5; 26 3.275,-1; 27 3.275,-0.5; 28 3.275,0; 29 3.275,0.5; 30 3.275,1; 31 3.275,1.5; 32 3.275,2; 33 3.275,2.5 | smd 0.275 x 0.75: 12 -2.5,-3.275; 13 -2,-3.275; 14 -1.5,-3.275; 15 -1,-3.275; 16 -0.5,-3.275; 17 0,-3.275; 18 0.5,-3.275; 19 1,-3.275; 20 1.5,-3.275; 21 2,-3.275; 22 2.5,-3.275; 34 2.5,3.275; 35 2,3.275; 36 1.5,3.275; 37 1,3.275; 38 0.5,3.275; 39 0,3.275; 40 -0.5,3.275; 41 -1,3.275; 42 -1.5,3.275; 43 -2,3.275; 44 -2.5,3.275 | smd 4.826 x 4.826: EXP 0,0
SOT23-DBV = smd 0.55 x 1.2: 1 -0.95,-1.3; 2 0,-1.3; 3 0.95,-1.3; 4 0.95,1.3; 5 -0.95,1.3
CRYSTAL-3.2-2.5 = smd 1.3 x 1.05: 1 -1.15,-0.925; 2 1.15,-0.925; 3 1.15,0.925; 4 -1.15,0.925
CT/CN0603 = smd 1 x 1: 1 -1,0; 2 1,0

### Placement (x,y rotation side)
ALS1_NM  119.61,51.56 0 top
C2  64.75,56.9 270 top
C3  54.08,56.9 270 top
C4  88.63,56.9 270 top
C5  99.29,56.9 270 top
C6  46.33,18.29 270 top
C7  89.51,15.24 0 top
C8  74.4,18.8 0 top
C9  64.37,29.46 0 top
C10  70.59,43.43 0 top
C11  70.59,37.34 180 top
C12  74.4,15.24 0 top
C13  89.64,34.54 0 top
C14  70.59,45.97 180 top
C15  98.28,48.51 90 top
C16  80.75,48.39 90 top
C17  89.64,43.94 0 top
C18  117.58,39.12 0 top
C19  74.4,29.46 0 top
C20  74.4,32 0 top
C21  89.64,25.91 180 top
C22  103.1,48.51 270 top
C23  64.37,26.16 180 top
C24  93.2,48.51 270 top
C25  64.37,18.8 180 top
C26  74.4,12.7 0 top
C27  49,25.65 270 top
C28  49,30.86 270 top
C29  25.38,8.38 90 top
C30  86.09,48.39 90 top
C31  78.47,48.39 90 top
C33  33.38,8.38 270 top
C34  30.84,8.38 270 top
C35  41.76,8.38 90 top
D1  36.3,8.38 90 top
DISCLAIMER  [DISC]  not placed on the board
F1  89.64,50.55 90 top
FID1  25.76,29.97 0 top
FID2  140.82,29.97 0 top
FID3  78.72,7.11 0 top
IC1  41.76,13.34 270 top
IC2  82.02,18.29 0 top
IC3  98.4,23.5 90 top
IC4  82.02,29.34 180 top
ICSP  63.99,50.29 90 top
INA  93.96,56.9 0 top
INB  104.63,56.9 0 top
J1  82.02,58.42 180 top
L  30.46,54.74 0 top
L1  95.74,48.51 90 top
L2  76.18,52.2 90 top
LCD1  82.02,33.78 90 top
LED1  112.25,6.86 0 top
LINEAR  82.02,7.11 0 top
ON  27.16,54.74 0 top
OUT2  59.42,56.9 0 top
OUT3  70.08,56.9 0 top
P1  29.95,29.97 90 top
PH1  119.87,51.56 90 top
PH2_NM  119.87,51.56 0 top
R1  46.46,13.97 90 top
R2  39.22,8.38 270 top
R3  28.3,8.38 90 top
R4  44.3,8.38 270 top
R5  49,13.97 90 top
R6  74.4,23.88 270 top
R7  73.39,52.2 270 top
R8  117.58,44.2 0 top
R9  74.27,40.39 0 top
R10  82.91,15.24 0 top
R11  117.58,41.66 180 top
R12  49,37.97 270 top
R13  69.07,23.88 90 top
R14  90.28,18.8 80 top
RN1  89.13,30.99 270 top
RN2  82.28,51.56 0 top
RN3  32.24,50.8 0 top
RN4  113.26,22.23 270 top
RX  37.06,54.74 0 top
S1  134.85,19.3 135 top
S2  124.19,29.97 225 top
S3  134.85,40.64 315 top
S4  145.78,29.97 225 top
SG1  44.43,51.56 90 top
SJ1  74.4,24.64 270 top
SJ2  69.07,24.64 270 top
T1  47.86,42.42 90 top
TS42  19.28,51.56 180 top
TX  33.76,54.74 0 top
U1  51.67,6.99 90 top
U2  82.02,39.88 270 top
U4  64.37,22.1 270 top
Y1  70.34,40.39 0 top
Z1  78.47,52.2 270 top
Z2  86.09,52.2 270 top

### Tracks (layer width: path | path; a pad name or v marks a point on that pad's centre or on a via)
+3V3
  Top 0.279: IC4.6 80.01,30.35 79.23,30.35 79.23,29.34
  Top 0.305: SJ1.1 75.93,26.16 79.1,29.34 79.23,29.34 IC4.7
  Top 0.406: SJ2.1 69.58,26.16 69.58,26.29
  Top 0.61: 66.02,26.29 66.02,28.57 65.26,29.34 C9.2 | U4.5 66.02,23.24 66.02,25.91 C23.+ 66.02,26.29 | 66.02,26.29 69.58,26.29 74.27,26.29 SJ1.1
+5V  (via drill 0.61)
  Top 0.279: U2.34 85.68,37.38 87.25,36.78 v87.76,36.29 87.86,36.47 87.86,36.45 | U2.2 84.02,44.04 84.69,44.7 84.69,46.1 C30.1 86.21,47.5 | U2.7 81.52,45.36 80.78,46.1 80.57,46.1 79.18,47.5 C31.1 | U2.14 78.19,41.38 77.93,41.12 75.95,41.12 75.42,41.66 75.16,41.66 74.4,42.42 73.64,42.42 72.62,43.43 72.62,44.83 C14.1 | C13.1 88.63,34.67 | RN4.4 111.67,21.02 111.61,21.08 | RN4.1 111.8,23.43 | 111.8,23.43 111.61,23.37 111.61,23.36 111.8,23.43 | RN4.2 111.63,22.62 111.61,22.61 | RN4.3 111.72,21.82 111.61,21.72
  Top 0.305: C6.2 45.32,17.4 44.18,16.26 44.18,14.35 44.14,14.31 IC1.8 | RN3.3 32.64,49.64 32.75,49.53 33.38,49.53 33.44,49.59 RN3.4
  Top 0.406: v39.22,10.67 R2.1 | 63.35,20.95 U4.3 62.97,21.13 61.83,21.13 61.45,21.51 61.45,22.71 61.83,23.09 63,23.09 U4.1 | 93.45,16.51 IC3.24 92.05,16.51 90.78,15.24 C7.2 v90.4,17.02 90.4,17.4 R14.1 | v30.71,48.51 30.71,49.66 RN3.1 | v33.76,48.51 33.76,49.66 RN3.4 | v115.3,45.21 R8.1 | 70.27,53.02 70.72,53.09 R7.1 | C2.2 66.65,56.01 OUT3.3 | OUT2.3 55.99,56.01 C3.2 | C24.2 93.2,47.37 | v94.85,38.1 94.85,44.96 v95.74,45.85 | 87.86,36.45 87.86,36.32 | 87.86,36.32 87.86,35.43 88.63,34.67 | v87.76,36.29 87.76,36.43 87.86,36.32 | C6.2 v47.99,17.4 | 111.61,21.08 111.61,21.72 111.61,22.61 111.61,23.36 | 111.61,23.37 111.61,24.13 110.85,24.89 LCD1.9
  Top 0.61: v27.41,15.88 P1.V1 v27.41,27.43 | 63.35,20.95 63.35,19.05 C25.2 63.35,18.67 v63.35,17.14 | v76.94,18.8 C8.2 v75.29,17.14 | v59.16,16.51 60.3,15.37 60.3,9.14 LINEAR.1 | v41.51,54.86 v41.51,48.51 | C3.2 53.32,56.01 52.94,55.63 v52.94,54.86 53.26,54.55 56.05,54.55 58.4,52.2 58.4,49.91 v57.76,49.28 | C22.+ 103.23,45.85 103.48,45.21 104.75,46.48 107.42,46.48 LCD1.1 | C14.1 v71.48,48.64 70.34,49.78 70.34,52.7 70.27,53.02 v70.34,53.09 | v76.94,48.01 77.2,48.01 77.7,47.5 C31.1 | INB.3 102.09,56.01 C5.2 99.29,55.24 99.04,54.99 v99.04,54.1 | INA.3 90.4,56.01 C4.2 | 89.9,48.77 F1.1 | INA.3 91.42,54.86 92.18,54.1 92.18,50.42 90.4,48.64 | 91.42,56.77 INA.3 | 88.37,48.39 88.75,48.77 89.51,48.77 F1.1 | C30.1 v84.56,48.01 | v95.74,45.85 L1.1 95.74,47.62 C24.2 91.42,47.62 90.4,48.64 | C2.2 63.73,54.99 v63.73,54.48 66.4,54.48 v67.8,53.09 | v33.76,48.51 v33.76,27.43 | 90.4,48.64 89.69,48.64 F1.1 | v112.5,37.59 112.5,42.42 v115.3,45.21
  Bottom 0.406: v33.76,48.51 v30.71,48.51 | v94.85,38.1 94.59,37.85 92.82,37.85 90.78,39.88 89.13,39.88 87.86,38.61 87.86,36.66 v87.76,36.29 | 47.99,13.21 v47.99,17.4
  Bottom 0.61: v27.41,15.88 27.41,11.94 28.68,10.67 v39.22,10.67 41.76,13.21 47.99,13.21 55.86,13.21 v59.16,16.51 59.8,17.14 v63.35,17.14 v75.29,17.14 75.67,16.76 79.48,16.76 79.86,16.38 89.77,16.38 v90.4,17.02 | v27.41,27.43 v33.76,27.43 P1.H1 | IC2.1 79.1,18.29 78.59,18.8 v76.94,18.8 | v41.51,48.51 v33.76,48.51 | v41.51,54.86 44.18,54.86 SG1.+ 44.56,54.86 v52.94,54.86 53.32,54.48 v63.73,54.48 | v57.76,49.28 59.29,47.75 ICSP.2 | v115.3,45.21 LCD1.1 107.42,45.21 106.28,44.07 105.01,44.07 103.87,45.21 100.06,45.21 99.42,45.85 v95.74,45.85 | v71.48,48.64 74.27,48.64 74.91,48.01 v76.94,48.01 v84.56,48.01 86.21,49.66 86.21,51.69 INA.3 91.42,56.39 93.71,54.1 v99.04,54.1 | v70.34,53.09 v67.8,53.09 | LCD1.9 110.72,24.89 112.5,26.67 v112.5,37.59
A4  (via drill 0.61)
  Top 0.279: v93.45,39.24 91.55,41.15 89.26,41.15 88.49,40.38 U2.40 | v99.67,38.61 99.67,36.58 100.18,36.07 100.18,33.02 99.17,32 99.17,21.34 98.79,20.95 98.79,19.68 101.96,16.51 IC3.1
  Bottom 0.279: v93.45,39.24 93.83,39.62 95.36,39.62 96.37,38.61 v99.67,38.61
A-LIGHT  (via drill 0.61)
  Top 0.305: v100.18,20.32 IC3.4 | v118.98,20.32 118.98,21.59 118.22,22.35 118.22,24.77 119.61,26.16 119.61,30.86 118.47,32 C18.2 R11.1 119.36,41.66 121.65,43.94 121.65,50.04 120.36,51.32 ALS1_NM.2
  Top 0.406: PH1.2 120.36,52.77 ALS1_NM.2 PH2_NM.2
  Bottom 0.305: v100.18,20.32 106.15,20.32 106.91,19.56 110.22,19.56 110.85,20.19 116.18,20.19 116.57,19.81 118.47,19.81 v118.98,20.32
A-LINEAR  (via drill 0.61)
  Top 0.305: v75.29,8 C26.2 83.8,12.7 85.58,14.48 v85.58,20.7 | v101.33,21.72 103.23,21.72 IC3.5
  Bottom 0.305: v75.29,8 73.64,6.35 63.73,6.35 62.72,5.33 60.56,5.33 LINEAR.2 | v85.58,20.7 89.51,20.7 90.53,21.72 v101.33,21.72
A-MIC  (via drill 0.61)
  Top 0.305: IC3.2 104.75,17.78 105.52,17.02 v105.52,14.99 | R3.1 C34.2 C33.2 34.65,7.49 35.16,6.86 36.17,6.86 D1.C v36.3,4.95
  Bottom 0.305: v36.3,4.95 37.95,4.95 42.02,9.02 55.99,9.02 58.53,11.56 60.56,11.56 63.48,14.48 77.2,14.48 77.83,13.84 79.35,13.84 79.99,14.48 95.99,14.48 98.02,16.51 99.29,16.51 100.69,14.99 v105.52,14.99
A-S1  (via drill 0.61)
  Top 0.279: RN4.7 114.9,22.62 115.93,21.59 115.93,20.95 118.22,18.67 124.18,18.67 S1.P$3 128.07,22.16 v129.39,20.83 | S1.P$4 138.09,12.52 138.03,12.57
  Top 0.305: v138.03,19.05 138.03,12.57 | IC3.9 104.75,26.67 105.26,26.16 105.26,24.13 106.41,22.99 106.41,21.72 108.06,20.07 110.72,20.07 v112.37,18.41
  Bottom 0.305: v138.03,19.05 137.01,19.05 135.11,20.95 129.52,20.95 v129.39,20.83 126.73,18.16 115.93,18.16 115.42,18.67 112.63,18.67 v112.37,18.41
A-S2  (via drill 0.61)
  Top 0.279: 117.23,26.72 S2.P$1 117.35,26.67 117.33,26.67
  Top 0.305: v127.49,31.75 127.49,36.58 S2.P$2 | v117.33,29.97 117.33,27.05 S2.P$1 | 117.33,26.67 v117.33,21.34 115.24,23.43 RN4.8 | v101.2,25.53 103.31,25.53 IC3.8
  Bottom 0.305: v117.33,29.97 121.9,29.97 123.68,31.75 v127.49,31.75 | v101.2,25.53 102.98,25.53 104.88,23.62 104.88,21.84 105.39,21.34 106.41,21.34 107.29,20.45 109.83,20.45 110.34,20.95 116.18,20.95 116.57,21.34 v117.33,21.34
A-S3  (via drill 0.61)
  Top 0.279: RN4.5 114.46,21.02 114.66,20.83 114.66,18.16 113.9,17.4 111.74,17.4 109.83,19.3 107.42,19.3 105.77,20.95 105.77,22.73 104.37,24.13 IC3.7 | S3.P$4 131.42,47.24 | 141.71,37.72 141.71,37.46 S3.P$3
  Top 0.305: IC3.7 100.69,24.13 99.93,24.89 99.93,26.29 100.06,26.42 100.06,31.75 100.94,32.64 100.94,42.16 102.6,43.81 104.25,43.81 v105.64,45.21 | v128.5,47.37 131.04,47.37 131.42,47.24 | v141.71,47.24 141.71,37.72
  Bottom 0.305: v141.71,47.24 v128.5,47.37 107.04,47.37 106.53,46.86 106.53,46.1 v105.64,45.21
A-S4  (via drill 0.61)
  Top 0.279: RN4.6 114.81,21.82 115.3,21.34 115.3,17.91 114.15,16.76 111.36,16.76 109.45,18.67 v105.9,18.67 | S4.P$3 142.52,22.94 142.6,22.86 | S4.P$4 152.63,33.15
  Top 0.305: IC3.6 104.63,22.86 105.14,22.35 105.14,19.81 105.9,19.05 v105.9,18.67 | 142.6,22.86 v142.6,20.57 | v152.63,20.57 152.63,33.15
  Bottom 0.305: v105.9,18.67 110.6,18.67 111.36,19.43 115.8,19.43 116.18,19.05 125.71,19.05 128.63,21.97 135.49,21.97 136.89,20.57 v142.6,20.57 v152.63,20.57
A-TEMP  (via drill 0.61)
  Top 0.305: C12.2 v78.72,15.24 R10.1 IC2.2 | v101.33,18.92 103.36,18.92 103.43,19 IC3.3
  Bottom 0.305: v78.72,15.24 95.61,15.24 99.29,18.92 v101.33,18.92
AREF
  Top 0.279: U2.42 87.71,41.38 88.75,42.42 90.15,42.42 90.53,42.8 C17.2
AVCC  (via drill 0.61)
  Top 0.279: v87.1,43.43 85.83,43.43 85.32,42.93 85.32,42.41 U2.44 | U2.24 80.02,35.59 79.1,34.67
  Top 0.305: 79.1,34.67 79.1,34.16 | 95.99,49.53 96.63,49.53 97.64,48.51 97.64,48.26 C15.1
  Top 0.406: 79.1,34.16 v78.47,33.78 | v98.28,34.04 98.28,35.31 97.13,36.45 v97.13,40.26 97.13,44.32 98.28,45.47 C15.1 98.02,47.5 | L1.2 95.99,49.53
  Bottom 0.279: 74.91,32.38 75.49,32.97 77.65,32.97
  Bottom 0.406: v87.1,43.43 89.64,43.43 92.44,40.64 95.74,40.64 96.12,40.26 v97.13,40.26 | v98.28,34.04 96.75,32.51 92.69,32.51 91.42,33.78 87.74,33.78 86.72,32.77 86.59,32.77 84.56,30.73 75.67,30.73 74.91,31.5 74.91,32.38 | 77.65,32.97 v78.47,33.78
BUZZ-CMD  (via drill 0.61)
  Top 0.305: U2.27 81.52,33.92 v81.39,33.78 | R12.2 49,34.8 49.38,34.42 52.3,34.42 52.94,33.78 65.64,33.78 v66.4,34.54
  Bottom 0.279: 77.32,35.31 76.05,34.04 66.91,34.04 v66.4,34.54
  Bottom 0.305: 77.32,35.31 79.86,35.31 v81.39,33.78
D7/LCD_CS  (via drill 0.61)
  Top 0.279: U2.1 84.53,43.53 86.97,45.97
  Top 0.305: 86.97,45.97 86.97,46.1 87.86,46.99 91.04,46.99 91.8,46.23 93.71,46.23 v93.96,45.97
  Bottom 0.305: LCD1.5 110.22,35.05 110.85,35.69 110.85,42.93 109.83,43.94 107.42,43.94 106.79,43.31 104.37,43.31 103.23,44.45 99.29,44.45 98.91,44.83 95.1,44.83 v93.96,45.97
D+
  Top 0.356: 82.02,54.1 81.01,53.09
  Top 0.381: J1.P3 82.02,54.1
  Top 0.406: Z1.1 78.47,53.09 81.01,53.09 81.02,53.09 81.08,53.03 RN2.8
D-
  Top 0.381: J1.P2 82.68,53.95 83.48,53.16 RN2.5
  Top 0.406: 86.09,53.21 86.09,53.09 83.53,53.09 83.48,53.16
  Top 0.61: Z2.1 86.09,53.21
G-SEL
  Top 0.305: IC4.10 81.62,27.73 81.11,27.22 78.25,27.22 75.67,24.64 SJ1.2 R6.1
GND  (via drill 0.61)
  Top 0.203: U2.23 79.52,37.25 80.12,37.85
  Top 0.254: 79.53,36.61 79.53,36.14 79.02,35.64 | 79.53,36.63 79.53,36.61 | 79.53,36.61 U2.23 | 85.22,37.87 U2.35 | 85.32,37.87 85.78,37.87 87.03,37.74 | 38.59,12.37 40.54,12.37 40.8,12.12
  Top 0.279: U2.5 82.52,41.78 | 82.52,41.78 82.52,40.89 | 82.52,40.89 82.52,40.38 U2.EXP 82.02,37.85 | U2.15 82.51,40.88 82.52,40.89 | 82.52,41.78 82.62,41.88 U2.43 86.43,41.88 86.85,42.29 | 82.02,37.85 82.05,37.88 U2.35 85.32,37.87 | 80.12,37.85 82.02,37.85 | IC4.5 80.82,30.92 80.37,31.37
  Top 0.305: 82.62,41.88 83.58,41.88 v83.8,41.66
  Top 0.381: J1.P5 80.7,54.18 80.62,54.1
  Top 0.406: IC3.16 93.32,26.67 93.34,26.63 | IC3.17 93.32,25.53 93.41,25.53 | 63.1,22.1 64.37,22.1
  other vias: 90.28,50.55 88.5,50.55 84.56,49.91 79.86,51.94 101.07,53.21 145.78,29.97 134.85,40.64 134.85,19.3 124.19,29.97 19.28,51.56 112.25,6.86 44.43,51.56 41.76,10.92 80.62,24.77 86.21,24.77 116.06,24.51 116.18,16.64 100.69,46.61 105.64,48.01
  pour Bottom (isolate 0.305, rank 2): 165.08,60.96 -2.56,60.96 -2.56,-2.54 165.08,-2.54
  pour Top (isolate 0.305, rank 2): -5.1,63.5 167.62,63.5 167.62,-5.08 -5.1,-5.08
HWB
  Top 0.279: U2.33 85.8,36.6 86.92,35.49 86.92,33.59 87.7,32.81 RN1.1
INA  (via drill 0.61)
  Top 0.305: v100.18,51.18 100.18,47.88 99.42,47.12 99.42,45.34 98.4,44.32 98.4,36.58 99.42,35.56 99.42,33.4 97.26,31.24 97.26,29.72 96.63,29.08 96.63,27.43 97.64,26.42 97.64,22.1 97.26,21.72 97.26,19.05 95.99,17.78 IC3.23 | v94.47,51.82 94.47,54.74 93.96,55.24 INA.2
  Bottom 0.305: v94.47,51.82 99.55,51.82 v100.18,51.18
INB
  Top 0.305: INB.2 104.63,55.24 103.61,54.23 100.69,54.23 97.9,51.44 95.86,51.44 94.72,50.29 94.72,48.9 95.1,48.51 96.63,48.51 97.13,48.01 97.13,45.72 95.74,44.32 95.74,39.62 96.12,39.24 96.12,35.31 96.88,34.54 96.88,33.15 96.37,32.64 96.37,29.97 95.86,29.46 95.86,26.92 96.88,25.91 96.88,22.48 96.5,22.1 96.5,19.43 96.12,19.05 IC3.22
IO8/CARD_CS  (via drill 0.61)
  Top 0.279: U2.28 82.02,34.54 87.99,28.57
  Top 0.305: 87.99,28.57 v87.99,27.43
  Top 0.406: v104.25,32.51 LCD1.6
  Bottom 0.305: v87.99,27.43 89.26,26.16 98.15,26.16 104.25,32.26 v104.25,32.51
IO11/DC_LCD  (via drill 0.61)
  Top 0.279: U2.20 77.6,38.38 v76.69,37.47
  Bottom 0.279: 86.21,44.83 85.7,44.32 80.62,44.32 80.12,43.81 76.56,43.81 76.05,43.31 76.05,42.29 76.43,41.91 76.43,38.61 76.69,38.35 v76.69,37.47 | 90.28,43.94 92.69,41.53 97.77,41.53 98.15,41.15 101.71,41.15 104.75,38.1 104.75,36.2 106.91,34.04 106.91,30.35 107.29,29.97
  Bottom 0.305: 86.21,44.83 88.24,46.86 89.64,46.86 90.15,46.35 90.15,44.07 90.28,43.94
  Bottom 0.406: 107.29,29.97 LCD1.7
IO13  (via drill 0.61)
  Top 0.279: U2.32 84.02,36.05 85.02,35.05 v85.7,35.05
  Top 0.305: v32.24,43.94 32.24,49.02 31.84,49.42 RN3.2
  Bottom 0.279: 76.89,35.89 75.6,34.59 68.1,34.59 67.14,35.56 67.04,35.56
  Bottom 0.305: v32.24,43.94 50.65,44.07 53.45,46.86 56.24,46.86 57.89,45.21 57.89,41.4 63.73,35.56 67.04,35.56 | v85.7,35.05 81.51,35.05 80.68,35.89 76.89,35.89
J-SW  (via drill 0.61)
  Top 0.305: v91.04,20.32 IC3.21 | v51.03,18.29 50.27,19.05 50.27,24.38 49.89,24.77 C27.2 v46.46,24.77
  Top 0.406: R14.2 91.04,20.2 v91.04,20.32
  Bottom 0.305: v46.46,24.77 19.28,24.77 P1.B1A | v91.04,20.32 90.15,19.43 85.07,19.43 83.55,20.95 76.56,20.95 73.89,18.29 v51.03,18.29
J-XOUT  (via drill 0.61)
  Top 0.305: C29.2 25.38,10.03 29.95,14.61 P1.V2 | 93.45,21.59 IC3.20 94.85,21.59 95.61,22.35 v95.61,23.11
  Bottom 0.305: P1.V2 29.95,21.08 30.59,21.72 34.65,21.72 35.79,20.57 52.94,20.57 53.7,19.81 73.13,19.81 76.31,22.99 89.13,22.99 90.4,24.26 91.67,24.26 92.82,23.11 v95.61,23.11
J-YOUT  (via drill 0.61)
  Top 0.305: v46.46,29.97 C28.2 51.16,29.97 51.54,29.59 51.54,23.37 51.16,22.99 51.16,20.45 v52.18,19.43 | v91.04,22.86 IC3.19
  Bottom 0.305: P1.H2 v46.46,29.97 | v91.04,22.86 90.28,22.86 89.39,21.97 76.43,21.97 73.51,19.05 52.56,19.05 v52.18,19.43
LED-B
  Top 0.279: U2.29 82.53,34.92 87.67,29.79 RN1.4
LED-G
  Top 0.279: U2.30 83.02,35.32 87.76,30.59 RN1.3
LED-R
  Top 0.279: U2.31 83.52,35.71 87.84,31.39 RN1.2
MISO  (via drill 0.61)
  Top 0.279: v73.64,47.37 75.29,45.72 75.29,44.7 76.18,43.81 79.23,43.81 79.52,43.52 U2.11
  Bottom 0.305: 104.25,42.42 102.98,43.69 99.04,43.69 98.66,44.07 94.21,44.07 92.56,45.72 92.56,47.12 90.28,49.4 87.74,49.4 85.07,46.74 84.05,46.74 83.8,46.99 77.83,46.99 77.7,46.86 76.31,46.86 76.18,46.99 74.02,46.99 v73.64,47.37 71.1,47.37 70.72,47.75 ICSP.1
  Bottom 0.406: 104.25,42.42 107.17,42.42 107.42,42.67 LCD1.2
MOSI  (via drill 0.61)
  Top 0.254: 63.99,49.02 v63.99,44.83
  Top 0.279: U2.10 80.02,43.83 79.41,44.45 77.2,44.45 v76.69,44.96
  Top 0.305: ICSP.4 63.99,49.02
  Bottom 0.305: v63.99,44.83 67.29,44.83 67.92,45.47 75.42,45.47 75.8,45.09 76.56,45.09 v76.69,44.96 77.2,44.45 79.48,44.45 80.24,45.21 85.7,45.21 88.37,47.88 89.51,47.88 90.78,46.61 90.78,45.47 93.71,42.55 97.77,42.55 98.15,42.16 101.96,42.16 106.53,37.59 107.55,37.59
  Bottom 0.406: 107.17,37.59 107.55,37.59 LCD1.4
MUXA  (via drill 0.61)
  Top 0.279: U2.36 87.13,38.38 88.88,37.85 v90.15,36.7 | v102.21,36.32 101.71,35.81 101.71,32.26 100.82,31.37 100.82,28.96 101.96,27.94 IC3.10
  Bottom 0.279: v90.15,36.7 90.91,35.94 96.63,35.94 97.01,36.32 v102.21,36.32
MUXB  (via drill 0.61)
  Top 0.279: U2.37 87.47,38.88 89.39,38.48 v89.9,38.48 | v103.48,37.59 103.48,35.56 102.47,34.54 102.47,31.88 101.58,30.99 101.58,29.59 101.96,29.21 IC3.11
  Bottom 0.279: v89.9,38.48 90.66,38.48 92.31,36.83 96.12,36.83 96.5,37.21 101.2,37.21 101.58,37.59 v103.48,37.59
MUXC  (via drill 0.61)
  Top 0.279: v93.07,33.78 93.07,36.96 90.4,39.62 89.51,39.62 89.27,39.38 U2.38 | v95.48,33.78 95.48,30.35 94.98,29.84 94.98,29.46 94.72,29.21 IC3.14
  Bottom 0.279: v93.07,33.78 v95.48,33.78
MUXD
  Top 0.279: IC3.13 94.09,30.48 94.09,36.96 90.66,40.39 89.39,40.39 88.88,39.88 U2.39
N$1
  Top 0.305: 38.59,13.66 36.89,13.66 36.3,13.08 D1.A 36.3,9.91 | 38.59,13.66 39.17,13.66 IC1.2 | IC1.1 38.67,14.31 38.59,14.22 38.59,13.66
N$2
  Top 0.305: RN3.7 31.84,52.31 L.A
N$3
  Top 0.305: RN3.8 31.09,51.44 30.33,52.2 29.7,52.2 28.17,53.72 27.41,53.72 ON.A
N$4  (via drill 0.61)  (1 unrouted)
  Top 0.305: IC4.13 84.02,27.4 83.55,26.92 82.02,26.92 81.51,26.42 80.37,26.42 v78.72,24.77 | v70.85,24.77 R13.2
  Bottom 0.305: v78.72,24.77 v70.85,24.77
N$6
  Top 0.305: RN3.6 32.64,52.31 TX.A
N$8
  Top 0.305: RN3.5 33.38,51.44 34.14,52.2 34.78,52.2 36.3,53.72 37.32,53.72 RX.A
N$11  (via drill 0.61)
  Top 0.279: RN1.7 90.55,31.39
  Top 0.305: 90.55,31.39 v91.04,31.88 | v82.53,24.77 83.8,23.5 84.43,23.5 86.85,21.08 86.85,20.19 86.47,19.81 86.47,7.49 v89.64,4.32 | v110.22,10.92 110.22,9.03 LED1.1
  Bottom 0.305: v91.04,31.88 89.51,31.88 88.63,30.99 87.74,30.99 86.72,29.97 86.72,28.7 84.82,26.8 84.56,26.8 v82.53,24.77 | v89.64,4.32 92.05,4.32 93.71,5.97 100.94,5.97 101.83,5.08 108.44,5.08 110.22,6.86 v110.22,10.92
N$12  (via drill 0.61)
  Top 0.279: RN1.6 90.55,30.59 v91.04,30.1
  Top 0.305: v84.31,24.77 87.74,21.34 87.74,19.81 87.36,19.43 87.36,9.14 v89.64,6.86 | v108.18,6.86 LED1.2
  Bottom 0.305: v89.64,6.86 101.33,6.86 102.21,5.97 107.17,5.97 108.06,6.86 v108.18,6.86 | v91.04,30.1 88.12,30.1 87.48,29.46 87.48,28.45 85.45,26.42 85.45,25.91 v84.31,24.77
N$13  (via drill 0.61)
  Top 0.279: RN1.5 89.81,28.49 v89.77,28.45
  Top 0.305: v97.9,28.45 97.9,27.43 98.4,26.92 98.4,21.72 98.02,21.34 98.02,17.27 98.66,16.64 v98.66,15.24 | v107.42,10.92 107.42,8.76 106.41,7.75 106.41,5.33 107.17,4.57 110.09,4.57 LED1.3
  Bottom 0.305: v107.42,10.92 106.15,12.19 105.14,12.19 103.23,14.1 99.8,14.1 v98.66,15.24 | v89.77,28.45 v97.9,28.45
N$17
  Top 0.305: SG1.- 44.43,42.93 45.06,42.29 46.46,42.29 T1.3
N$19  (via drill 0.61)
  Top 0.305: R2.2 C35.1 v41.76,4.95
  Bottom 0.305: v41.76,4.95 50.27,4.95 U1.1
N$20
  Top 0.305: C35.2 R4.1 44.3,10.79 43.92,11.18 43.92,12.32 IC1.5
N$21
  Top 0.305: R5.1 R1.1 46.39,13.01 IC1.6
N$23
  Top 0.305: IC1.3 39.52,13.01 42.17,13.01 42.83,13.66 IC1.7 45.01,13.66 46.21,14.86 R1.2
N$27
  Top 0.305: R8.2 118.47,45.34 119.87,46.74 PH1.1
  Top 0.406: PH2_NM.1 ALS1_NM.1 118.86,50.87 PH1.1
N$31
  Top 0.305: R12.1 49,41.15 T1.1
OUT2  (via drill 0.61)
  Top 0.279: v60.18,42.42 60.18,54.74 59.42,55.5 OUT2.2 | U2.12 77.49,42.38 v77.07,42.8
  Bottom 0.279: 71.99,36.2 72.37,36.58 75.93,36.58 76.05,36.45 77.32,36.45 77.7,36.83 77.7,38.61 77.07,39.24 v77.07,42.8 | 64.11,37.47 60.18,41.4 v60.18,42.42
  Bottom 0.305: 71.99,36.2 68.31,36.2 67.42,37.08 64.5,37.08 64.11,37.47
OUT3  (via drill 0.61)
  Top 0.279: U2.18 76.31,39.38 75.29,38.35 v74.4,38.35
  Top 0.305: v66.53,38.35 66.53,43.18 67.92,44.58 67.92,47.12 67.67,47.37 67.67,51.05 69.07,52.45 69.07,53.85 70.08,54.86 OUT3.2
  Bottom 0.305: v74.4,38.35 74.02,38.35 73.39,37.72 67.16,37.72 v66.53,38.35
RD+
  Top 0.279: U2.4 83.02,44.47 82.91,44.58
  Top 0.305: 82.91,44.58 82.91,46.48 81.89,47.5 81.89,49.78 81.08,50.35 RN2.1
RD-
  Top 0.279: U2.3 83.52,44.68 83.8,44.96
  Top 0.305: 83.8,44.96 83.8,46.61 82.71,47.7 82.71,48.95 83.48,49.71 RN2.4
RESET  (via drill 0.61)
  Top 0.279: U2.13 77.8,41.88 77.67,41.75 76.26,41.75 75.6,42.42 75.42,42.42 74.66,43.18 74.02,43.18 73.39,43.81 73.39,45.72 72.5,46.61 72.5,48.01 72.62,48.13 72.62,49.53 71.73,50.42 v71.73,51.31 R7.2
  Top 0.305: TS42.2 15.22,49.15 v19.28,49.15 23.22,49.15 TS42.1 | v49.76,56.9 v49.76,46.23
  Bottom 0.305: v71.73,51.31 66.78,51.31 ICSP.5 65.77,53.34 65.77,55.88 64.75,56.9 64.75,57.78 63.61,58.93 51.8,58.93 v49.76,56.9 | v49.76,46.23 22.2,46.23 v19.28,49.15
RST_LCD  (via drill 0.61)
  Top 0.279: U2.21 78.12,37.88 77.83,37.59 77.83,37.08 77.2,36.45 75.8,36.45 75.54,36.7 73.51,36.7
  Top 0.305: 73.51,36.7 71.61,34.8 v71.61,31.5
  Bottom 0.305: v71.61,31.5 71.61,31.24 73,29.84 84.94,29.84 87.36,32.26 87.99,32.26 88.88,33.02 91.29,33.02 92.69,31.62 100.69,31.62 103.1,34.04 105.14,34.04 105.9,33.27 105.9,28.32 106.79,27.43
  Bottom 0.406: 106.79,27.43 LCD1.8
RXLED  (via drill 0.61)
  Top 0.279: U2.8 81.02,44.71 79.25,46.48 77.58,46.48 77.2,46.86 76.31,46.86 75.54,47.62 v75.54,49.28
  Top 0.305: RX.C 38.68,55.79 v38.71,55.75
  Bottom 0.279: v75.54,49.28 75.04,49.66 70.46,49.66 69.7,49.02 64.5,49.02 63.99,48.51 63.99,46.99 63.48,46.48 59.03,46.48 56.88,48.64 53.83,48.64 49.76,52.7 49,52.7
  Bottom 0.305: 49,52.7 40.37,52.7 38.71,54.36 v38.71,55.75
SCK  (via drill 0.61)
  Top 0.279: U2.9 80.52,44.27 79.33,45.47 v78.59,45.47
  Top 0.305: ICSP.3 66.27,50.29 66.78,49.78 v66.78,46.23
  Bottom 0.305: 105.39,40.13 102.6,42.93 98.66,42.93 98.28,43.31 93.96,43.31 91.67,45.59 91.67,46.86 89.9,48.64 88.12,48.64 85.45,45.97 83.42,45.97 83.29,46.1 79.23,46.1 v78.59,45.47 78.08,45.97 76.05,45.97 75.8,46.23 v66.78,46.23
  Bottom 0.406: 105.39,40.13 LCD1.3
TXLED  (via drill 0.61)
  Top 0.254: U2.22 78.63,37.38
  Top 0.279: 78.63,37.38 78.63,36.62 77.83,35.81 77.07,35.81
  Top 0.305: 77.07,35.81 75.29,35.81 v75.04,35.56 | TX.C 35.25,55.79 v35.29,55.75
  Bottom 0.279: 63.86,36.58 58.65,41.78 58.65,45.59 56.49,47.75 53.32,47.75 50.78,50.29 43.16,50.29 42.78,50.67 38.59,50.67
  Bottom 0.305: 38.59,50.67 35.29,53.98 v35.29,55.75 | v75.04,35.56 68.05,35.56 67.29,36.32 64.11,36.32 63.86,36.58
UCAP
  Top 0.279: U2.6 82.02,46.23 C16.1
USH  (via drill 0.61)
  Top 0.406: J1.S6 81.13,58.29 83.04,58.29 J1.S5
  Top 0.813: J1.S6 J1.S2 J1.S4 79.43,55.75 77.58,55.75 76.18,54.36 L2.2 | J1.S5 J1.S6 | J1.S6 J1.S1 J1.S3
  other vias: 77.45,55.75 86.59,55.75 82.02,57.4
  pour Top (isolate 0.406): 76.94,61.98 87.1,61.98 87.1,55.24 76.94,55.24
  pour Bottom (isolate 0.406): 76.94,61.98 87.1,61.98 87.1,55.24 76.94,55.24 76.94,61.85
XOUT  (via drill 0.61)
  Top 0.279: IC4.2 83.22,31.18 83.54,31.5 84.18,31.5 85.7,29.97 85.7,29.59 | C21.2 86.47,25.91 85.7,26.67 v85.7,29.08 | U2.41 88.1,40.88 89.01,41.78 91.55,41.78 92.69,42.93 92.69,44.07 90.53,46.23 89.26,46.23 v88.88,45.85
  Top 0.305: v85.7,29.08 85.7,29.59
  Bottom 0.279: 77.65,34.75 76.41,33.5 71.46,33.5 71.23,33.27
  Bottom 0.305: v85.7,29.08 85.58,29.21 72.24,29.21 70.46,30.99 v70.46,32.64 71.23,33.27 | 77.65,34.75 79.02,34.75 81.01,32.77 85.45,32.77 87.23,34.54 87.23,35.31 86.47,36.07 86.47,42.29 85.96,42.8 85.96,43.69 87.86,45.59 88.63,45.59 v88.88,45.85
XTAL1
  Top 0.279: U2.17 76.05,39.88 75.54,39.37 73.39,39.37
  Top 0.305: R9.1 73.39,39.37 73.39,38.61 72.12,37.34 C11.1 69.58,39.24 69.32,39.24 Y1.1
XTAL2
  Top 0.279: U2.16 75.3,40.38 R9.2
  Top 0.305: 71.61,41.53 71.48,41.66 | 71.48,41.66 C10.2 | 71.61,41.53 Y1.3 71.61,41.15 71.61,41.53 | 71.48,41.66 74.02,41.66 75.04,40.64 R9.2
XUSB
  Top 0.381: J1.P1 83.34,54.69 83.55,54.61
  Top 0.61: F1.2 88.71,52.5 87.1,54.48 85.45,54.48 84.94,54.36 84.05,54.36 83.55,54.61
YOUT  (via drill 0.61)
  Top 0.279: U2.26 81.02,35.07 80.37,34.42 80.37,33.15 81.01,32.51 81.51,32.51 v82.28,31.75 82.42,31.6 IC4.3
  Top 0.305: C20.2 v76.43,32
  Bottom 0.305: v76.43,32 77.2,32 77.45,31.75 v82.28,31.75
ZOUT
  Top 0.279: U2.25 80.52,35.33 79.74,34.54 79.74,32.89 80.12,32.51 80.52,32.11 | 80.52,32.11 81.62,31.01 IC4.4 | C19.2 76.43,29.46 78.97,32 80.42,32 80.52,32.11

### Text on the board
Bottom: 2012-REV04
tPlace: Prototype | Limited | Edition | BUZZER | LIGHT | RESET | ACCEL | Y | SELF-T | Z | X | 6g | 1.5 | TEMP | MICRO | LED
tNames: M.Banzi | D.Cuartielles | T.Igoe | G.Martino | D.Mellis | 1 | TM | Arduino | Esplora | arduino.cc
bNames: MADE IN | ITALY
